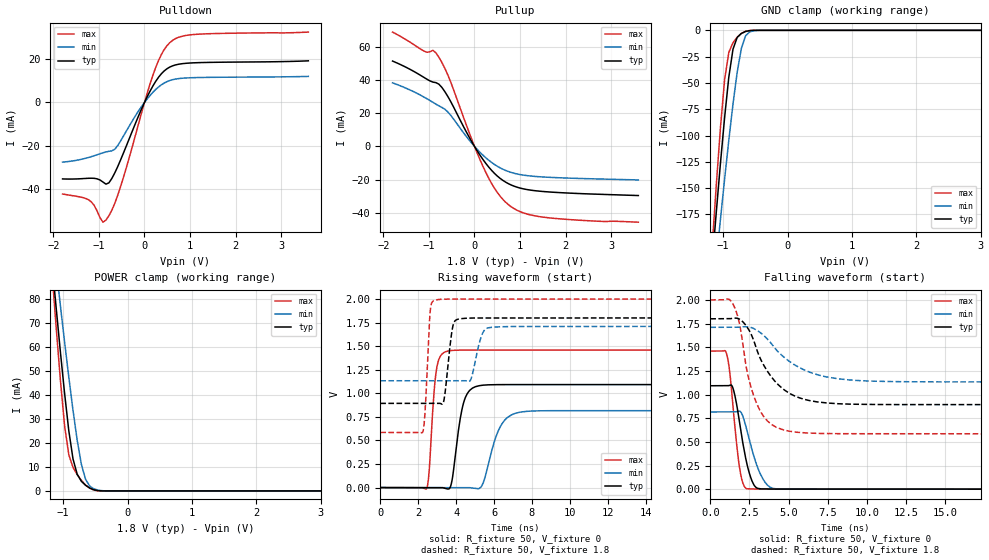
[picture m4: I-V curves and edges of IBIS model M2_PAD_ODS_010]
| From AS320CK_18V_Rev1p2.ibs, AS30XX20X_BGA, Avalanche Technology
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[Model] M2_PAD_ODS_010
Model_type I/O
Enable   Active-High
Vinl  =  0.63
Vinh  =  1.17
Vmeas =  0.9
Cref  =  30e-12
| Capacitance  typ   min   max
C_comp   1.624629e-12   1.520611e-12   1.744819e-12
| Variables   typ   min   max
[GND Clamp Reference]   0   0   0
[POWER Clamp Reference]   1.8   1.71   2
[Pulldown Reference]   0   0   0
[Pullup Reference]   1.8   1.71   2
[Temperature Range]   25   125   -40
[Voltage Range]   1.8   1.71   2
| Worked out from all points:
|   slope of the pulldown table from 0 to 0.27 V, typ, clamps not added: 25.7 ohm
|   slope of the pullup table from 0 to 0.27 V, typ, clamps not added: 24.7 ohm
|   GND clamp passes 1 mA (typ) near -0.64 V on its own axis
|   POWER clamp passes 1 mA (typ) near -0.57 V on its own axis
|   falling waveform, R_fixture 50, V_fixture 0: 20-80 % time 706ps typ, 900ps min, 524ps max; typ from 1.09 V to 0 V
|   falling waveform, R_fixture 50, V_fixture 1.8: 20-80 % time 1.87ns typ, 2.55ns min, 1.16ns max; typ from 1.8 V to 0.893 V
|   rising waveform, R_fixture 50, V_fixture 0: 20-80 % time 477ps typ, 754ps min, 290ps max; typ from 0 V to 1.09 V
|   rising waveform, R_fixture 50, V_fixture 1.8: 20-80 % time 292ps typ, 399ps min, 203ps max; typ from 0.893 V to 1.8 V
[GND Clamp]
| Voltage   I(typ)   I(min)   I(max)
-1.8V     -720.4mA   -670.5mA   -825.2mA
-1.173V   -222.3mA   -260.3mA   -207.5mA
-1.108V   -173.8mA   -219.8mA   -148.3mA
-1.043V   -126.9mA   -180.1mA   -93.11mA
-977.6mV  -83.02mA   -141.5mA   -47.01mA
-912.4mV  -44.68mA   -104.6mA   -21.04mA
-847.2mV  -17.95mA   -70.1mA    -11.75mA
-782.1mV  -6.736mA   -39.85mA   -6.526mA
-716.9mV  -2.917mA   -17.13mA   -2.96mA
-651.7mV  -1.107mA   -5.246mA   -907.6uA
-456.2mV  -3.886uA   -74.14uA   -373.5nA
3.6V      0A         0A         0A
[POWER Clamp]
| Voltage   I(typ)   I(min)   I(max)
-1.8V     287.1mA    268.3mA    329.6mA
-1.173V   94.89mA    108.5mA    91.02mA
-1.108V   76.1mA     92.66mA    67.97mA
-1.043V   57.9mA     77.16mA    46.14mA
-977.6mV  40.62mA    62.05mA    27.14mA
-912.4mV  25.13mA    47.46mA    15.06mA
-847.2mV  13.38mA    33.64mA    9.853mA
-716.9mV  4.014mA    11.09mA    4.394mA
-651.7mV  2.34mA     4.821mA    2.483mA
-586.6mV  1.18mA     2.003mA    1.113mA
-325.9mV  1.153uA    19.85uA    110.1nA
3.6V      0A         0A         0A
[Pulldown]
| Voltage   I(typ)   I(min)   I(max)
-1.8V     -35.5mA    -27.69mA   -42.5mA
-1.238V   -35.21mA   -25.6mA    -45.07mA
-912.4mV  -36.94mA   -23.37mA   -55.58mA
-847.2mV  -37.92mA   -22.98mA   -54.63mA
-716.9mV  -35.27mA   -22.46mA   -50mA
-521.4mV  -26.49mA   -17.75mA   -38.78mA
-65.17mV  -3.048mA   -1.907mA   -4.891mA
248.3mV   9.844mA    6.047mA    16.33mA
434.5mV   14.66mA    9.037mA    24.58mA
620.7mV   17.01mA    10.57mA    28.86mA
1.179V    18.47mA    11.56mA    31.67mA
3.6V      19.32mA    12.09mA    32.66mA
[Pullup]
| Voltage   I(typ)   I(min)   I(max)
-1.8V     51.33mA    38.22mA    68.75mA
-1.108V   41.45mA    29.65mA    57.3mA
-912.4mV  38.66mA    26.5mA     57.78mA
-782.1mV  37.42mA    24.38mA    53.62mA
-586.6mV  30.08mA    20.75mA    43.03mA
-65.17mV  3.06mA     2.09mA     4.59mA
248.3mV   -10.19mA   -6.826mA   -15.61mA
496.6mV   -17.7mA    -11.86mA   -27.5mA
744.8mV   -22.4mA    -15.09mA   -35.02mA
1.055V    -25.41mA   -17.19mA   -39.79mA
1.49V     -27.08mA   -18.35mA   -42.46mA
3.6V      -29.55mA   -20.16mA   -45.58mA
[Ramp]
dV/dt_r   0.655597/0.476918n  0.489635/0.75417n  0.875432/0.290065n
dV/dt_f   0.544074/1.87057n  0.346028/2.55295n  0.848876/1.15854n
R_load = 50
[Falling Waveform]
R_fixture = 50
V_fixture = 0
V_fixture_min = 0
V_fixture_max = 0
| Time   V(typ)   V(min)   V(max)
0s        1.093V     816.1mV    1.459V
1.052ns   1.093V     816.2mV    1.422V
1.251ns   1.097V     816.2mV    1.226V
1.438ns   1.072V     816.3mV    896.6mV
1.876ns   696.7mV    823.6mV    218.5mV
2.331ns   273.5mV    626.7mV    4.167mV
2.894ns   21.69mV    287.4mV    1.151mV
3.495ns   1.982mV    72.91mV    837.6uV
4.044ns   895.6uV    7.213mV    812.3uV
21.88ns   -2.321uV   906.9nV    -6.953uV
[Falling Waveform]
R_fixture = 50
V_fixture = 1.8
V_fixture_min = 1.71
V_fixture_max = 2
| Time   V(typ)   V(min)   V(max)
0s        1.8V       1.71V      2V
1.454ns   1.806V     1.711V     1.955V
1.823ns   1.8V       1.711V     1.78V
2.37ns    1.708V     1.716V     1.224V
2.755ns   1.577V     1.698V     995.7mV
3.431ns   1.304V     1.621V     762.3mV
4.221ns   1.124V     1.471V     653mV
5.692ns   964.8mV    1.284V     599.3mV
8.117ns   903.2mV    1.167V     586.4mV
21.88ns   893.2mV    1.133V     585.2mV
[Rising Waveform]
R_fixture = 50
V_fixture = 0
V_fixture_min = 0
V_fixture_max = 0
| Time   V(typ)   V(min)   V(max)
0s        1.933nV    49.93nV    1.563nV
2.448ns   -325uV     -312.3uV   -10.12mV
2.965ns   -393.6uV   -378.3uV   1.255V
3.533ns   -13.78mV   -450.7uV   1.447V
3.784ns   76.06mV    -482.7uV   1.455V
4.401ns   904.4mV    -561.5uV   1.459V
5.009ns   1.07V      -9.749mV   1.459V
6.326ns   1.092V     645.2mV    1.459V
7.129ns   1.093V     788.3mV    1.459V
21.88ns   1.093V     816.1mV    1.459V
[Rising Waveform]
R_fixture = 50
V_fixture = 1.8
V_fixture_min = 1.71
V_fixture_max = 2
| Time   V(typ)   V(min)   V(max)
0s        893.2mV    1.133V     585.2mV
2.244ns   893.9mV    1.134V     590.6mV
2.636ns   894mV      1.134V     1.876V
2.902ns   894.1mV    1.134V     1.989V
3.336ns   908mV      1.134V     1.999V
3.785ns   1.668V     1.134V     2V
4.117ns   1.787V     1.134V     2V
4.758ns   1.798V     1.14V      2V
5.739ns   1.799V     1.697V     2V
21.88ns   1.8V       1.71V      2V
